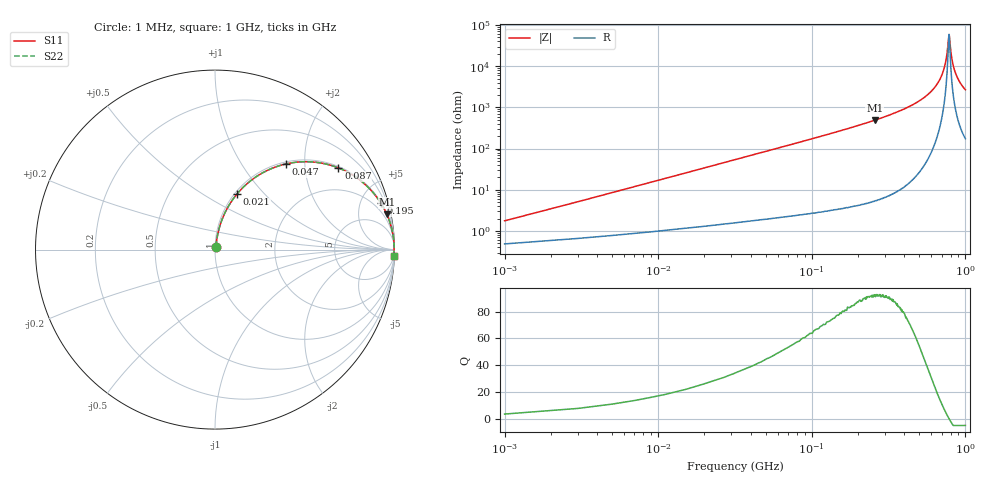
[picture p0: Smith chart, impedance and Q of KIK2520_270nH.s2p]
!version-2
!date-01.2022
!Series
# MHz S RI R 50
!Freq ReS11 ImS11 ReS21 ImS21 ReS12 ImS12 ReS22 ImS22
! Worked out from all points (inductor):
!   501 points, 1 MHz to 1 GHz, reference 50 ohm
!   read as one part in series: L = 270 nH near 5 MHz
!   highest Q = 91.8 at 257 MHz (marker M1), where L = 303 nH
!   self-resonance near 781 MHz
!   S11 on the Smith chart (normalised r, x): 1 MHz: 1.01, +0.03; 21 MHz: 1.03, +0.71; 47 MHz: 1.04, +1.60; 87 MHz: 1.05, +2.99; 195 MHz: 1.08, +7.05; 1 GHz: 4, -54
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1  0.00512 0.0168  0.9949 -0.0168  0.9949 -0.0168  0.00512 0.0168
7  0.0222 0.1151  0.9778 -0.1151  0.9778 -0.1151  0.0222 0.1151
9  0.0316 0.1465  0.9684 -0.1465  0.9684 -0.1465  0.0316 0.1465
15  0.0703 0.2339  0.9296 -0.2339  0.9296 -0.2339  0.0703 0.2339
21  0.1218 0.309  0.8782 -0.309  0.8782 -0.309  0.1218 0.309
47  0.393 0.4768  0.607 -0.4768  0.607 -0.4768  0.393 0.4768
87  0.6879 0.4551  0.3121 -0.4551  0.3121 -0.4551  0.6879 0.4551
169  0.8975 0.2972  0.1025 -0.2972  0.1025 -0.2972  0.8975 0.2972
195  0.923 0.2608  0.077 -0.2608  0.077 -0.2608  0.923 0.2608
257  0.9578 0.1956  0.0421 -0.1956  0.0421 -0.1956  0.9578 0.1956
335  0.9782 0.1404  0.0218 -0.1404  0.0218 -0.1404  0.9782 0.1404
501  0.9939 0.0689  0.00606 -0.0689  0.00606 -0.0689  0.9939 0.0689
667  0.998 0.0241  0.00202 -0.0241  0.00202 -0.0241  0.998 0.0241
709  0.9983 0.0149  0.00174 -0.0149  0.00174 -0.0149  0.9983 0.0149
739  0.9983 0.00865  0.00166 -0.00865  0.00166 -0.00865  0.9983 0.00865
757  0.9983 0.00504  0.00165 -0.00504  0.00165 -0.00504  0.9983 0.00504
777  0.9983 0.00113  0.00168 -0.00113  0.00168 -0.00113  0.9983 0.00113
783  0.9983 -2.86e-05  0.00169 2.86e-05  0.00169 2.86e-05  0.9983 -2.86e-05
809  0.9982 -0.00493  0.00179 0.00493  0.00179 0.00493  0.9982 -0.00493
835  0.9981 -0.00968  0.00193 0.00968  0.00193 0.00968  0.9981 -0.00968
899  0.9975 -0.0208  0.00248 0.0208  0.00248 0.0208  0.9975 -0.0208
1000  0.9962 -0.037  0.00379 0.037  0.00379 0.037  0.9962 -0.037
